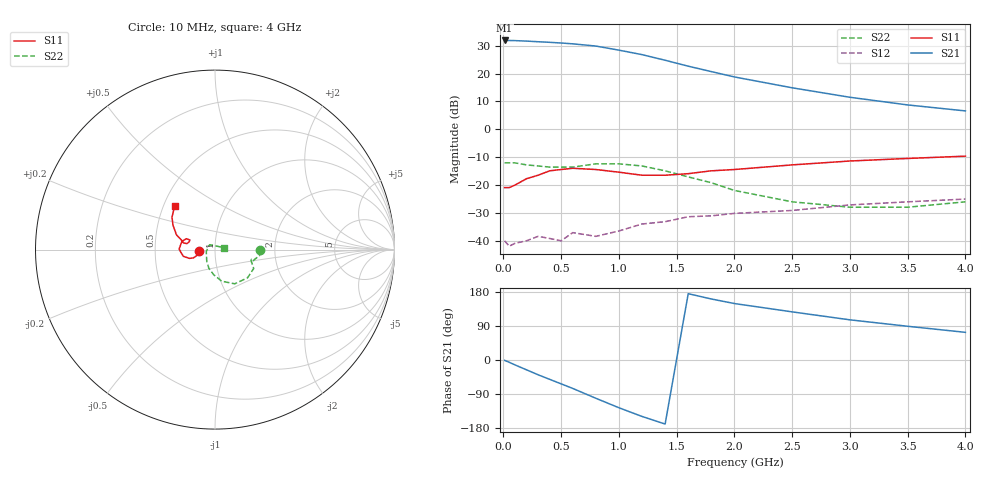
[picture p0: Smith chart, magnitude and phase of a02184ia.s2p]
!  INA-02184  S PARAMETERS
!  Id = 35 mA  LAST UPDATED 07-22-92
# ghz s ma r 50
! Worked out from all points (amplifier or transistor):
!   19 points, 10 MHz to 4 GHz, reference 50 ohm
!   highest |S21| = 31.9 dB at 10 MHz (marker M1)
!   |S21| within 3 dB of that: start of sweep to 935.2 MHz
!   unconditionally stable (mu >= 1): start of sweep to end of sweep
!   at 200 MHz: K = 1.44, MAG = 31.9 dB, |S12| = -40.0 dB
!   at 1 GHz: K = 1.40, MAG = 28.7 dB, |S12| = -36.5 dB
!   at 4 GHz: K = 3.75, MAG = 7.1 dB, |S12| = -25.0 dB
0.01  0.09 -176.0  39.33 -1.0  0.01 1.0  0.25 -1.0
0.05  0.09 -171.0  39.24 -6.0  0.008 -12.0  0.25 -4.0
0.1  0.1 -163.0  39.07 -13.0  0.009 1.0  0.25 -8.0
0.2  0.13 -159.0  38.3 -26.0  0.01 15.0  0.23 -13.0
0.3  0.15 -161.0  37.3 -39.0  0.012 16.0  0.22 -17.0
0.4  0.18 -168.0  36.42 -51.0  0.011 32.0  0.21 -15.0
0.5  0.19 -175.0  35.4 -63.0  0.01 34.0  0.21 -16.0
0.6  0.2 179.0  34.2 -75.0  0.014 35.0  0.21 -17.0
0.8  0.19 166.0  31.21 -101.0  0.012 38.0  0.24 -26.0
1  0.17 159.0  26.36 -126.0  0.015 53.0  0.24 -41.0
1.2  0.15 159.0  21.89 -149.0  0.02 56.0  0.22 -60.0
1.4  0.15 163.0  17.36 -169.0  0.022 62.0  0.18 -78.0
1.6  0.16 168.0  13.59 175.0  0.027 67.0  0.14 -93.0
1.8  0.18 168.0  10.86 161.0  0.028 61.0  0.11 -108.0
2  0.19 165.0  8.71 149.0  0.031 64.0  0.08 -125.0
2.5  0.23 159.0  5.56 127.0  0.035 56.0  0.05 -167.0
3  0.27 150.0  3.76 106.0  0.044 65.0  0.04 155.0
3.5  0.3 143.0  2.74 89.0  0.05 57.0  0.04 137.0
4  0.33 133.0  2.14 73.0  0.056 62.0  0.05 13.0
